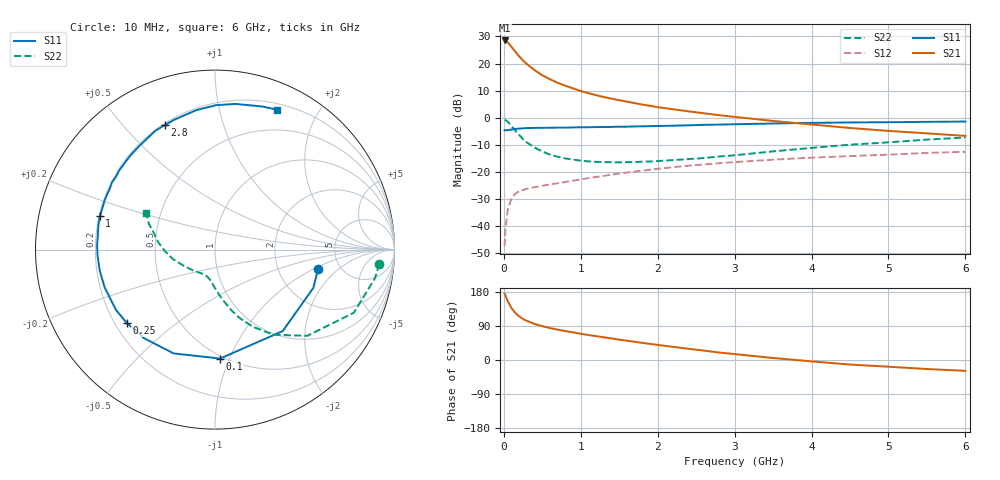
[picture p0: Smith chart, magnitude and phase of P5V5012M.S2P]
! SIEMENS Small Signal Semiconductors
! BFP183
! Si NPN RF Bipolar Junction Transistor in SOT143
! VCE = 0.5 V  IC = 12 mA
! Common Emitter S-Parameters:  March  1996
# GHz  S  MA  R  50
!  f  S11  S21  S12  S22
! GHz  MAG  ANG  MAG  ANG  MAG  ANG  MAG  ANG
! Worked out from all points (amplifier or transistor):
!   36 points, 10 MHz to 6 GHz, reference 50 ohm
!   highest |S21| = 28.5 dB at 10 MHz (marker M1)
!   |S21| within 3 dB of that: start of sweep to 117.5 MHz
!   unconditionally stable (mu >= 1): 667.4 MHz to end of sweep
!   at 250 MHz: K = 0.47, MSG = 23.8 dB, |S12| = -26.6 dB
!   at 1.4 GHz: K = 1.36, MAG = 10.4 dB, |S12| = -21.0 dB
!   at 6 GHz: K = 1.25, MAG = -0.1 dB, |S12| = -12.5 dB
!   S11 on the Smith chart (normalised r, x): 10 MHz: 3.42, -1.11; 100 MHz: 0.48, -0.93; 250 MHz: 0.25, -0.34; 1 GHz: 0.20, +0.14; 2.8 GHz: 0.21, +0.66; 6 GHz: 0.26, +1.50
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0.01  0.5844 -10.5  26.59 175.0  0.0043 85.5  0.9195 -5.0
0.02  0.588 -21.3  26.37 170.1  0.0086 82.1  0.9051 -10.2
0.05  0.5903 -50.3  24.63 155.5  0.02 69.9  0.8498 -24.4
0.1  0.6076 -87.3  20.25 136.8  0.0325 54.1  0.7042 -43.0
0.15  0.6227 -111.7  16.44 123.9  0.0403 44.9  0.5755 -55.5
0.2  0.6325 -128.7  13.51 114.7  0.0442 40.1  0.4784 -63.9
0.25  0.6391 -140.4  11.31 108.0  0.0468 36.5  0.404 -70.3
0.3  0.646 -148.5  9.749 103.2  0.049 35.6  0.3504 -74.8
0.4  0.6499 -161.0  7.527 95.1  0.0525 34.3  0.2826 -81.4
0.5  0.6529 -169.8  6.062 89.3  0.0558 34.8  0.2387 -86.5
0.6  0.6552 -176.9  5.13 84.3  0.0591 35.6  0.2096 -90.8
0.7  0.6574 177.9  4.403 80.2  0.062 36.7  0.1909 -94.2
0.8  0.6577 173.0  3.894 76.3  0.0654 37.4  0.1779 -97.0
1  0.6681 163.9  3.114 69.2  0.073 39.2  0.162 -102.8
1.1  0.6685 160.2  2.843 65.9  0.0774 39.5  0.1571 -105.8
1.5  0.6853 147.0  2.105 53.6  0.0938 40.4  0.1507 -115.9
2.2  0.714 126.7  1.435 34.7  0.1226 37.3  0.1658 -134.4
2.8  0.7484 111.8  1.115 19.7  0.1454 32.7  0.1932 -150.7
3.5  0.7839 97.7  0.873 5.3  0.169 26.9  0.2399 -167.2
4.5  0.8194 82.0  0.648 -12.0  0.1968 18.0  0.3191 172.6
5.5  0.841 71.2  0.516 -23.8  0.225 10.1  0.3954 158.7
6  0.8516 66.2  0.463 -28.6  0.2362 5.4  0.4335 152.2
